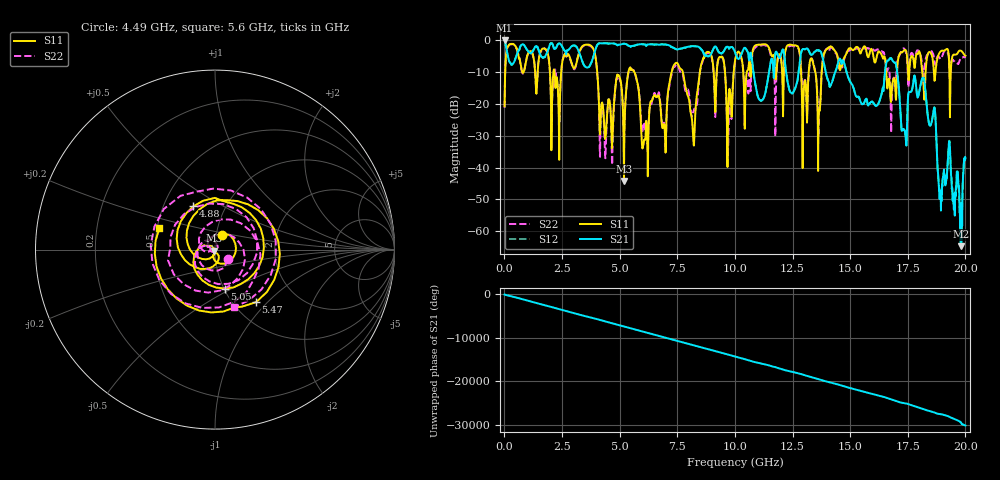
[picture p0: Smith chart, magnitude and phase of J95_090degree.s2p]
!Keysight Technologies,N5222A,MY51421036,A.10.65.16
!Date: Friday, March 31, 2023 14:17:20
!Correction: S11(Full 2 Port(1,2))
!S21(Full 2 Port(1,2))
!S12(Full 2 Port(1,2))
!S22(Full 2 Port(1,2))
!S2P File: Measurements: S11, S21, S12, S22:
# Hz S  dB  R 50
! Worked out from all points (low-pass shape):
!   2000 points, 10 MHz to 20 GHz, reference 50 ohm
!   highest |S21| = -0.11 dB at 10 MHz (marker M1); lowest = -64.7 dB at 19.8 GHz (marker M2)
!   |S21| within 3 dB of the highest: 1.896 GHz to 2.59 GHz (694.3 MHz wide, 31 % of centre); 3.945 GHz to 8.57 GHz (4.625 GHz wide, 73.9 % of centre)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
!   lowest |S11| = -44.2 dB at 5.19 GHz (marker M3), VSWR 1.01, Z = 49.7 - j0.539 ohm
!   |S11| at or under -10 dB: 4.027 GHz to 5.383 GHz (1.356 GHz wide, 28.8 % of centre); 5.635 GHz to 7.26 GHz (1.624 GHz wide, 25.2 % of centre); 7.74 GHz to 8.479 GHz (739.6 MHz wide, 9.12 % of centre)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
!   |S22| runs from -39.2 to -1.2 dB; largest |S21 - S12| = 0.014
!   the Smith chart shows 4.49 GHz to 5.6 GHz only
!   S11 on the Smith chart (normalised r, x): 4.49 GHz: 1.06, +0.18; 4.88 GHz: 0.71, +0.37; 5.05 GHz: 1.01, -0.46; 5.47 GHz: 1.27, -0.86; 5.6 GHz: 0.51, +0.14
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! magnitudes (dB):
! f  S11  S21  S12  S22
! 10 MHz  -20.8  -0.1  -0.1  -21.2
! 3.35 GHz  -2.2  -6.1  -6.1  -2.4
! 4.49 GHz  -20.8  -1.1  -1.0  -20.7
! 4.88 GHz  -11.4  -1.4  -1.4  -11.7
! 5.05 GHz  -13.0  -1.4  -1.3  -13.4
! 5.19 GHz  -44.2  -1.1  -1.1  -31.3
! 5.47 GHz  -8.6  -2.1  -2.0  -8.8
! 5.6 GHz  -9.6  -1.8  -1.8  -9.4
! 6.03 GHz  -32.8  -1.4  -1.3  -26.1
! 6.68 GHz  -17.3  -1.4  -1.4  -16.7
! 7.5 GHz  -7.2  -2.9  -2.9  -7.6
! 8.19 GHz  -30.4  -1.9  -1.9  -22.7
! 8.86 GHz  -3.7  -5.1  -5.1  -4.1
! 9.76 GHz  -15.3  -2.5  -2.5  -17.9
! 10.01 GHz  -6.2  -3.9  -3.9  -6.7
! 13.34 GHz  -5.9  -4.6  -4.6  -5.8
! 16.67 GHz  -12.2  -6.3  -6.3  -8.9
! 17.35 GHz  -3.1  -28.2  -28.3  -2.7
! 18.17 GHz  -12.9  -11.8  -11.7  -11.5
! 18.9 GHz  -3.7  -47.4  -47.8  -5.8
! 19.8 GHz  -3.3  -64.7  -59.5  -5.7
! 20 GHz  -4.9  -37.2  -37.0  -5.6
